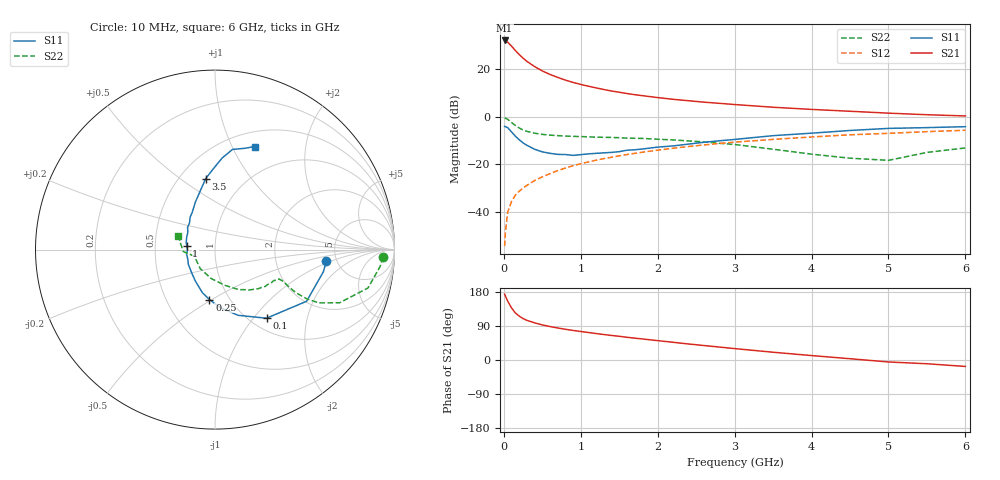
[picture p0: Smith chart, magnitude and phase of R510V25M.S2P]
! SIEMENS Small Signal Semiconductors
! BFR183
! Si NPN RF Bipolar Junction Transistor in SOT23
! VCE = 10 V  IC = 25 mA
! Common Emitter S-Parameters:  May  1996
# GHz  S  MA  R  50
!  f  S11  S21  S12  S22
! GHz  MAG  ANG  MAG  ANG  MAG  ANG  MAG  ANG
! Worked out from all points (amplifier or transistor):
!   36 points, 10 MHz to 6 GHz, reference 50 ohm
!   highest |S21| = 32.0 dB at 10 MHz (marker M1)
!   |S21| within 3 dB of that: start of sweep to 116.9 MHz
!   unconditionally stable (mu >= 1): 559.9 MHz to 2.572 GHz
!   at 250 MHz: K = 0.81, MSG = 27.3 dB, |S12| = -30.0 dB
!   at 1.4 GHz: K = 1.05, MAG = 12.6 dB, |S12| = -17.1 dB
!   at 6 GHz: K = 0.90, MSG = 3.0 dB, |S12| = -5.7 dB
!   S11 on the Smith chart (normalised r, x): 10 MHz: 4.12, -0.88; 100 MHz: 1.18, -1.17; 250 MHz: 0.81, -0.49; 1 GHz: 0.73, +0.03; 3.5 GHz: 0.67, +0.63; 6 GHz: 0.66, +1.23
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0.01  0.6243 -6.0  39.85 173.8  0.0019 78.0  0.9381 -2.6
0.02  0.6161 -11.6  39.11 168.9  0.0037 81.7  0.9244 -5.9
0.05  0.586 -29.4  36.61 155.5  0.0098 77.5  0.8786 -14.1
0.1  0.478 -53.1  30.34 137.3  0.0166 70.0  0.7549 -23.1
0.15  0.3883 -70.6  24.47 124.1  0.0224 68.5  0.6494 -27.2
0.2  0.3269 -84.3  20.17 115.8  0.0271 68.4  0.578 -28.2
0.25  0.2802 -96.4  16.92 109.3  0.0316 68.2  0.5251 -28.1
0.3  0.2498 -106.4  14.52 104.6  0.036 69.2  0.4911 -27.6
0.4  0.2064 -122.1  11.27 98.1  0.0454 70.3  0.4491 -26.3
0.5  0.182 -136.2  9.12 92.6  0.0544 71.0  0.4236 -25.2
0.6  0.1694 -151.3  7.697 88.3  0.0634 71.3  0.4083 -24.8
0.7  0.161 -159.8  6.678 84.5  0.0736 71.4  0.399 -24.7
0.8  0.1602 -170.7  5.859 81.1  0.0831 70.9  0.3908 -24.8
1  0.1592 172.0  4.75 75.2  0.1023 69.7  0.3812 -25.8
1.1  0.1651 166.3  4.356 72.5  0.1119 68.9  0.3763 -27.0
1.3  0.1736 154.6  3.71 67.2  0.1315 67.4  0.3676 -28.7
1.6  0.1971 140.8  3.059 59.9  0.16 64.3  0.3545 -32.9
2.2  0.2427 121.6  2.313 46.7  0.2167 58.1  0.3246 -42.2
3.5  0.3986 97.5  1.576 20.5  0.3326 41.8  0.207 -74.3
4.5  0.5122 85.5  1.297 3.4  0.4158 29.5  0.134 -127.9
5.5  0.5879 73.7  1.097 -9.9  0.4841 18.4  0.1773 -176.5
6  0.6156 68.9  1.034 -17.0  0.5174 11.1  0.22 159.2
